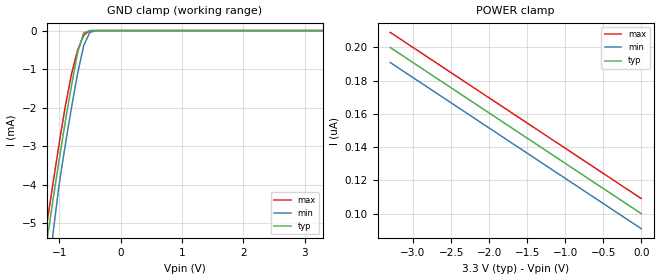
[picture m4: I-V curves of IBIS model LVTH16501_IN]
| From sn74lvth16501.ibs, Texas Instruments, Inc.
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|   LVTH16501 Input (IN) model
[Model]   LVTH16501_IN
Model_type  Input
Polarity   Non-Inverting
Vinl = 0.8V
Vinh = 2.0V
| variable   typ   min   max
C_comp   3.5p   NA   NA
[Temperature Range]   50   100   0
[Voltage range]   3.3   3   3.6
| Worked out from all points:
|   GND clamp passes 1 mA (typ) near -0.75 V on its own axis
|Process range|   weak   strong
[GND Clamp]
|   50C:3.3V:   100C:3V:weak   0C:3.6V:strong
|   Voltage   I(typ)   I(min)   I(max)
-3.3V     -75.35mA   -79.87mA   -70.95mA
-1.3V     -6.799mA   -9.477mA   -6.099mA
-1.2V     -5.468mA   -7.096mA   -5.007mA
-1.1V     -4.39mA    -5.263mA   -3.959mA
-1V       -3.353mA   -3.991mA   -2.929mA
-900mV    -2.358mA   -2.965mA   -1.962mA
-800mV    -1.44mA    -2.006mA   -1.138mA
-700mV    -574.5uA   -1.12mA    -511.4uA
-600mV    -59.21uA   -388uA     -117.9uA
-500mV    -1.902uA   -46.32uA   -901.7nA
-400mV    -64.81nA   -2.368uA   -24.86nA
3.3V      99.99nA    100nA      99.99nA
[POWER Clamp]
|   50C:3.3V:   100C:3V:weak   0C:3.6V:strong
|   Voltage   I(typ)   I(min)   I(max)
-3.3V     200nA      190.9nA    209.1nA
-2.8V     184.8nA    175.8nA    193.9nA
-2.1V     163.6nA    154.6nA    172.7nA
0V        99.99nA    90.93nA    109.1nA
